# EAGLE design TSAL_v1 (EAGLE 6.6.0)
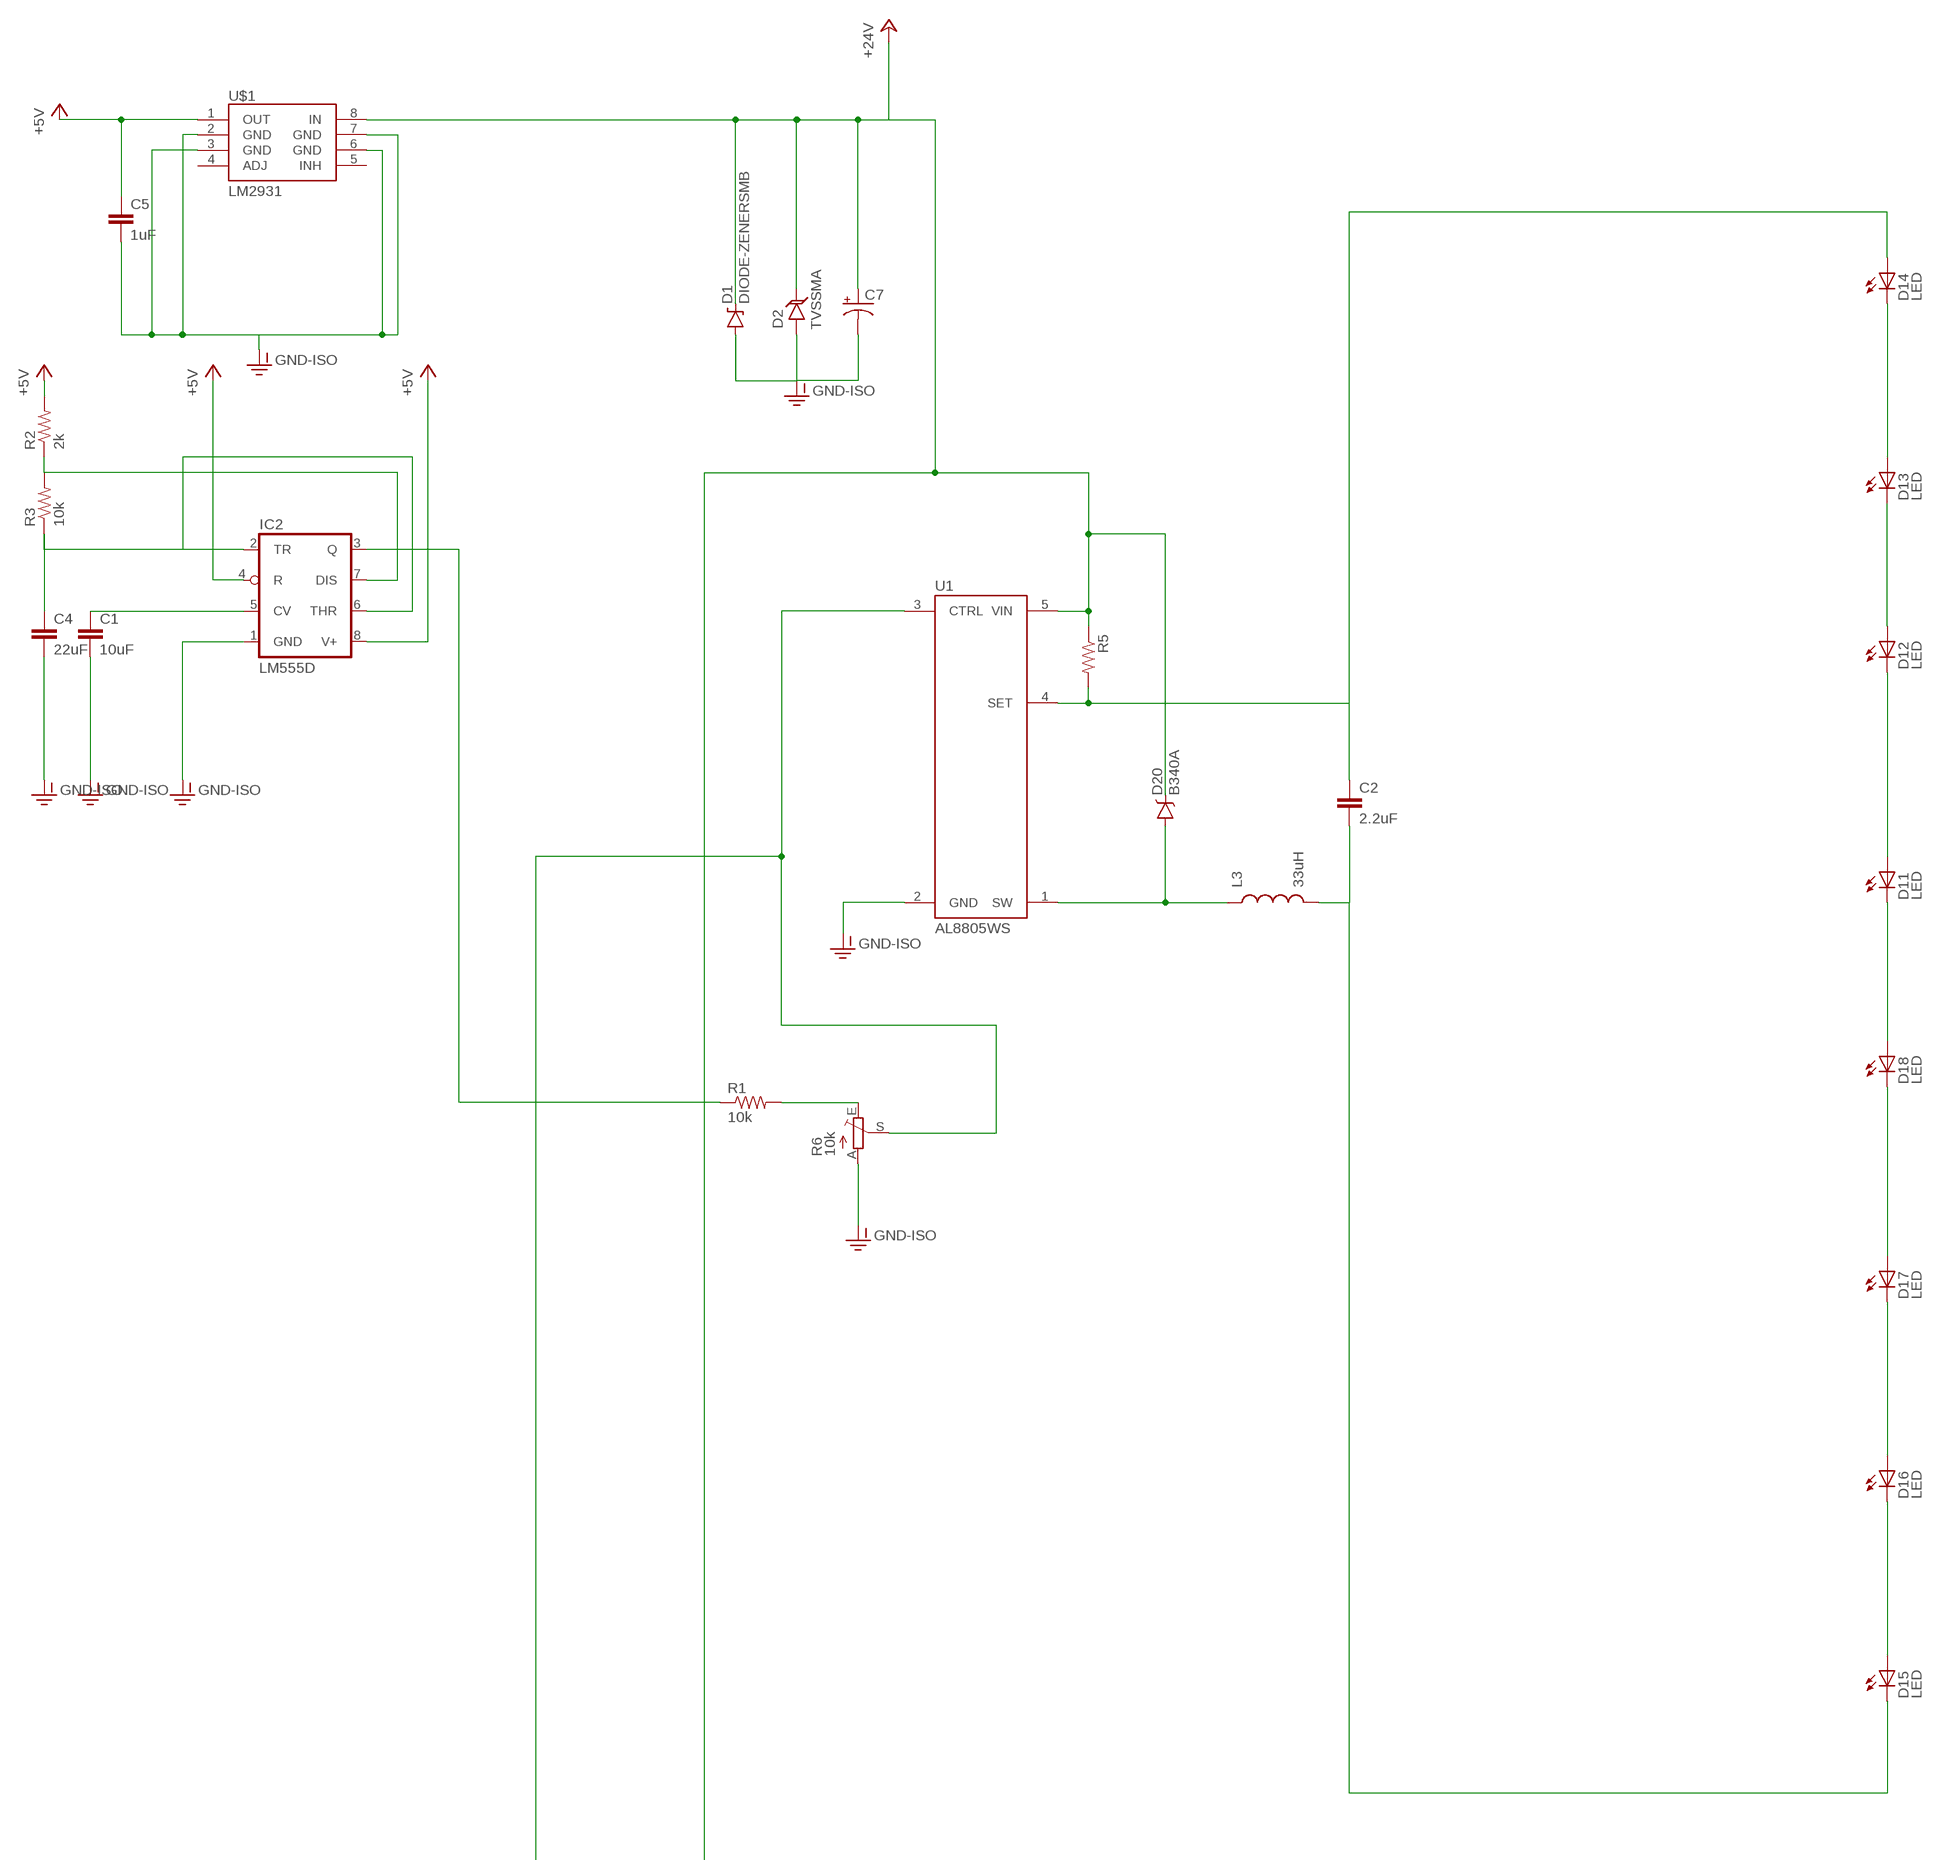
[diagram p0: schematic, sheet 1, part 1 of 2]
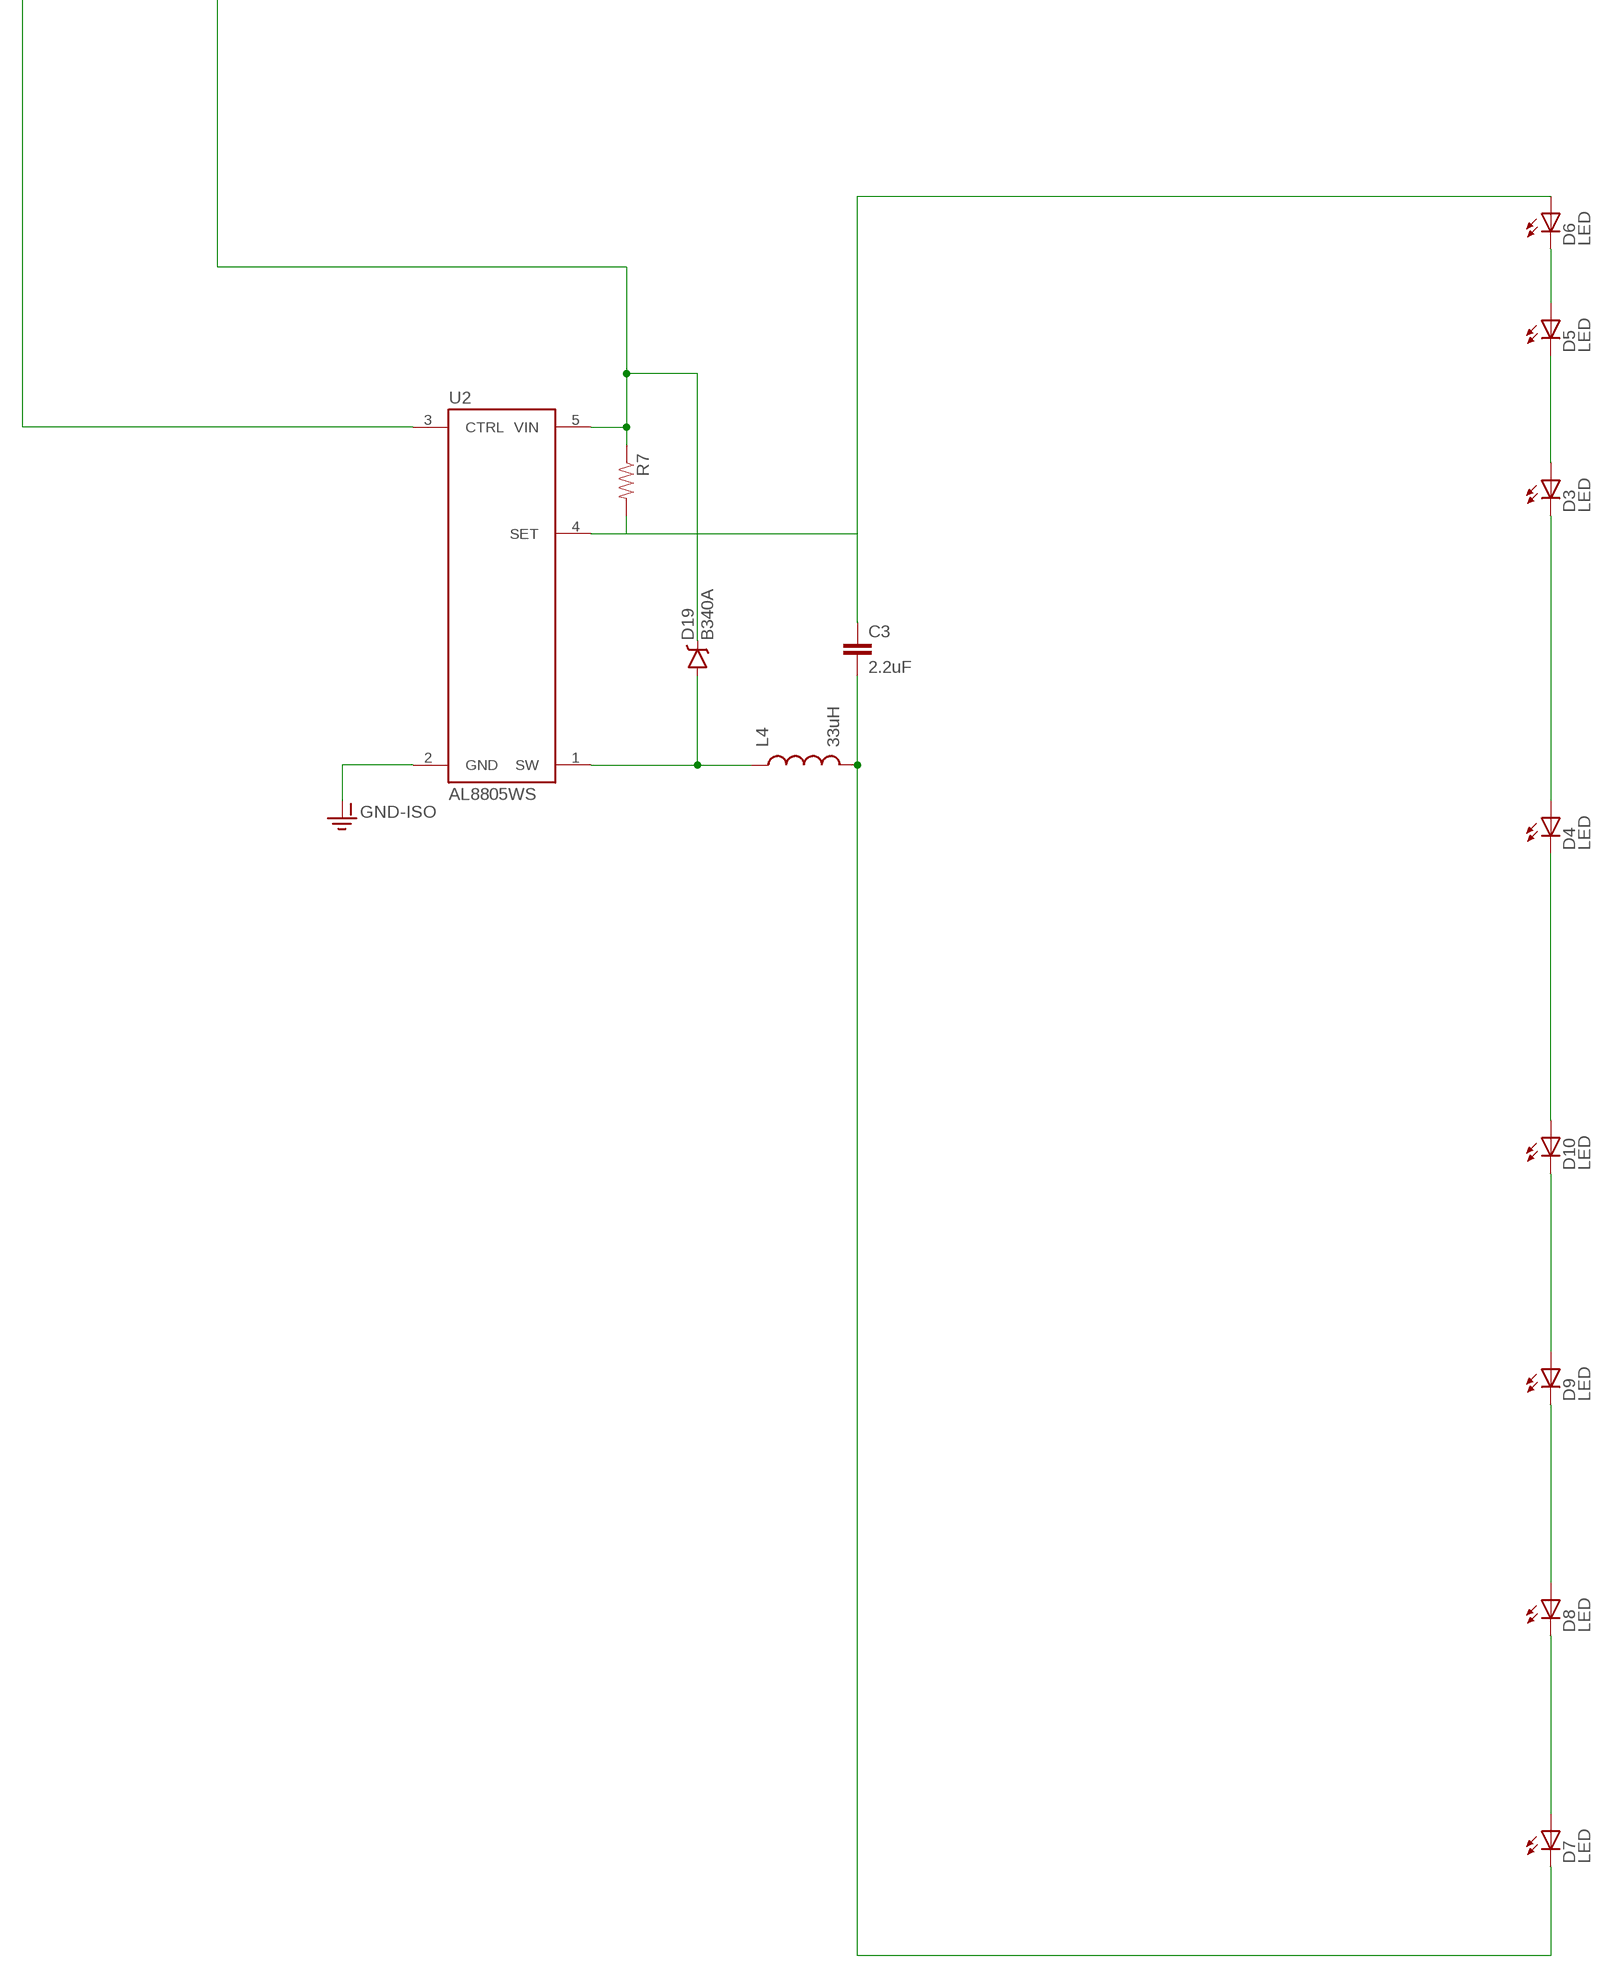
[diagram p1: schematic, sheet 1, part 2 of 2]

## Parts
C1  10uF  CAP0805  [0805]
C2  2.2uF  CAP0805  [0805]
C3  2.2uF  CAP0805  [0805]
C4  22uF  CAP0805  [0805]
C5  1uF  CAP0805  [0805]
C7  CAP_POL6032  [EIA6032]
D1  DIODE-ZENERSMB  [SMB-DIODE]
D2  TVSSMA  [SMA-DIODE]
D3  LED  [LED-SM]
D4  LED  [LED-SM]
D5  LED  [LED-SM]
D6  LED  [LED-SM]
D7  LED  [LED-SM]
D8  LED  [LED-SM]
D9  LED  [LED-SM]
D10  LED  [LED-SM]
D11  LED  [LED-SM]
D12  LED  [LED-SM]
D13  LED  [LED-SM]
D14  LED  [LED-SM]
D15  LED  [LED-SM]
D16  LED  [LED-SM]
D17  LED  [LED-SM]
D18  LED  [LED-SM]
D19  B340A  DIODE-SCHOTTKY-B340A  [SMA-DIODE]
D20  B340A  DIODE-SCHOTTKY-B340A  [SMA-DIODE]
IC2  LM555D  [SO08]
L3  33uH  INDUCTORBOURNS_SRN6045  [SRN6045]
L4  33uH  INDUCTORBOURNS_SRN6045  [SRN6045]
R1  10k  RESISTOR0805-RES  [0805]
R2  2k  RESISTOR0805-RES  [0805]
R3  10k  RESISTOR0805-RES  [0805]
R5  RESISTOR0805-RES  [0805]
R6  10k  TRIM_EU-B25P  [B25P]
R7  RESISTOR0805-RES  [0805]
U1  AL8805WS  AL8805  [SOT23-5]
U2  AL8805WS  AL8805  [SOT23-5]
U$1  LM2931  [SO08]

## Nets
+5V: C5.1 IC2.4(R) IC2.8(V+) R2.2 U$1.1(OUT)
+24V: C7.P$1(+) D1.C D2.C D19.C D20.C R5.1 R7.1 U1.5(VIN) U2.5(VIN) U$1.8(IN)
GND-ISO: C1.2 C4.2 C5.2 C7.P$2(-) D1.A D2.A IC2.1(GND) R6.A U1.2(GND) U2.2(GND) U$1.2(GND) U$1.3(GND) U$1.6(GND) U$1.7(GND)
N$1: C3.1 D6.A R7.2 U2.4(SET)
N$2: R6.S U1.3(CTRL) U2.3(CTRL)
N$3: D3.C D4.A
N$4: C1.1 IC2.5(CV)
N$5: IC2.7(DIS) R2.1 R3.2
N$6: IC2.3(Q) R1.1
N$7: D19.A L4.1 U2.1(SW)
N$8: C2.1 D14.A R5.2 U1.4(SET)
N$9: D13.A D14.C
N$10: C4.1 IC2.2(TR) IC2.6(THR) R3.1
N$11: D3.A D5.C
N$12: D12.A D13.C
N$13: D11.A D12.C
N$14: C3.2 D7.C L4.2
N$15: D11.C D18.A
N$16: D17.A D18.C
N$17: D5.A D6.C
N$18: D7.A D8.C
N$19: C2.2 D15.C L3.2
N$20: D8.A D9.C
N$21: D4.C D10.A
N$22: D9.A D10.C
N$23: D16.A D17.C
N$24: D15.A D16.C
N$26: D20.A L3.1 U1.1(SW)
N$27: R1.2 R6.E
Unconnected: U$1.4(ADJ) U$1.5(INH)

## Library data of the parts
C1-C5 = SparkFun-Capacitors:CAP: Capacitor
C7 = SparkFun-Capacitors:CAP_POL: Capacitor Polarized
D1 = SparkFun-DiscreteSemi:DIODE-ZENER: Zener Diode
D2 = SparkFun-DiscreteSemi:TVS: Transient voltage suppressor- prevents ESD on inputs.
D3-D18 = FSAE Eletric:LED
D19 D20 = SparkFun-DiscreteSemi:DIODE-SCHOTTKY: Schottky diodes in SFE's production catalog; PROD_ID: DIO-09886
IC2 = adafruit:*555: TIMER Changed DIP package to have round (not oval) pin pads http://www.ladyada.net/library/pcb/eaglelibrary.html
L3 L4 = SparkFun-Passives:INDUCTOR: Inductors; PROD_ID: NDUC-11627
R1-R3 R5 R7 = SparkFun-Passives:RESISTOR: Resistor
R6 = pot:TRIM_EU-: POTENTIOMETER
U1 U2 = SparkFun-PowerIC:AL8805: Constant current LED driver PWM-able 1MHz switch freq 6V-36V Up to 1A LED current; PROD_ID: IC-11626
U$1 = SparkFun-PowerIC:LM2931: LDO regulator with reverse battery protection- very durable!

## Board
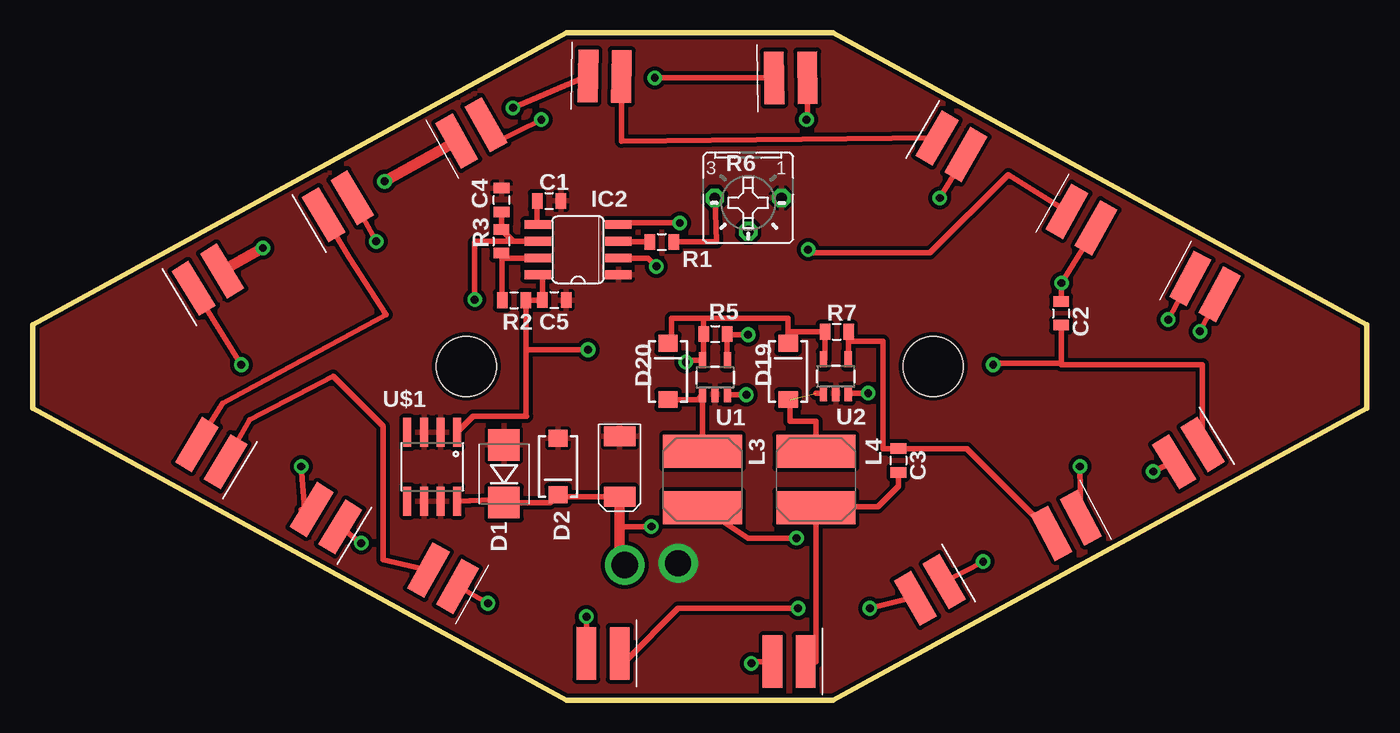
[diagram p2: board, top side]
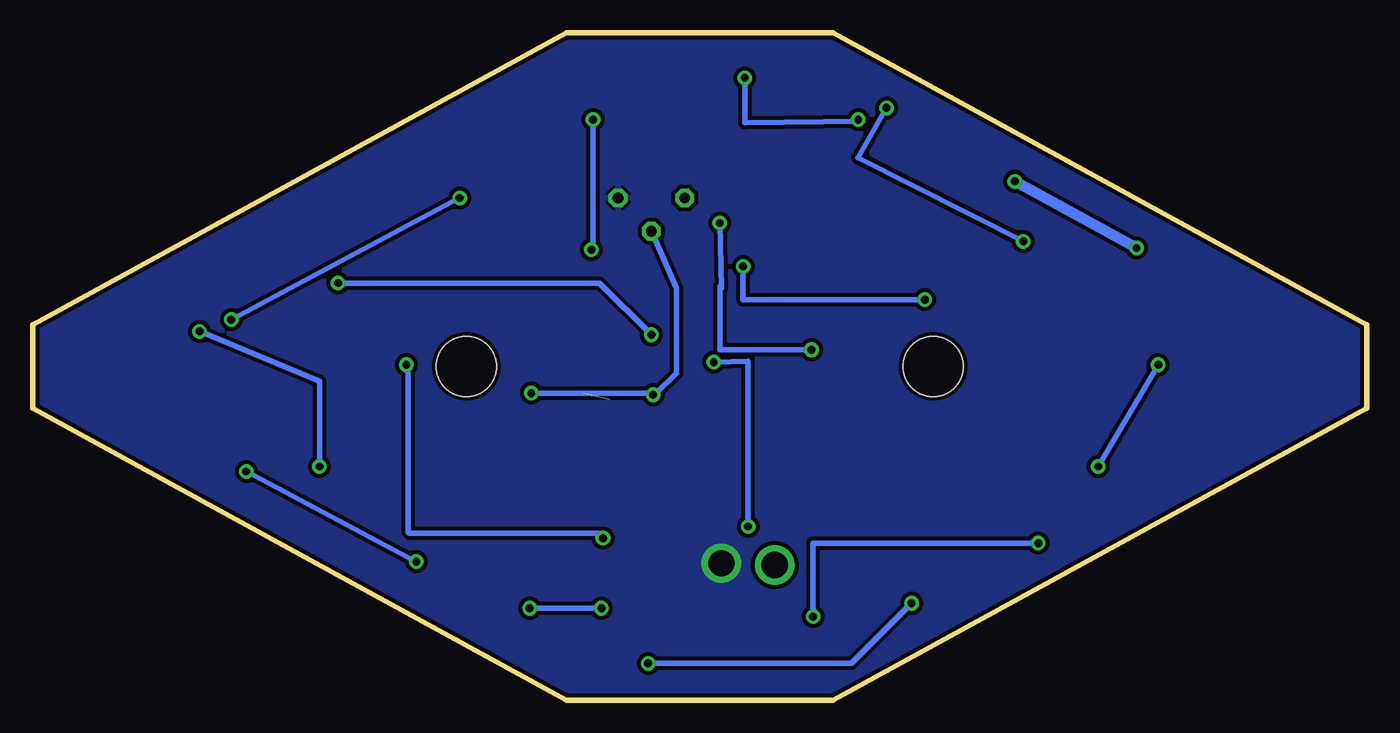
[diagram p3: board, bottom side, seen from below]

Size 101.6 x 50.8 mm. Coordinates in mm from the lower left corner, seen from the top.
Outline: 0,22.22 0,28.57 40.64,50.8 60.96,50.8 101.6,28.57 101.6,22.22 60.96,0 40.64,0 0,22.22
Copper layers (1*16): Top 0.035mm / dielectric 1.5mm / Bottom 0.035mm
Design rules "SparkFun": minimum track width 8mil, minimum drill 20mil, track to track 8mil, track to pad 8mil, pad to pad 8mil, via to via 8mil, smd to smd 8mil, copper to edge 10mil, drill to drill 8mil, minimum pad ring 12mil, minimum via ring 10mil, stop-mask expansion 4mil, vias tented up to drill 25mil, thermal gap 10mil
Holes 4.57 mm at 33.02,25.4 68.58,25.4

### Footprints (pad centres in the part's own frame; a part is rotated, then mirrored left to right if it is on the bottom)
0805 = smd 0.8 x 1.2: 1 -0.9,0; 2 0.9,0
EIA6032 = smd 1.5 x 2.4: P$1 -2.3,0; P$2 2.3,0
SMB-DIODE = smd 2.4 x 2.4: A 2.2,0; C -2.2,0
SMA-DIODE = smd 1.27 x 1.47: A -2.15,0; C 2.15,0
LED-SM = smd 1.5 x 4: A 1.27,0; C -1.27,0
SO08 = smd 0.66 x 2.032: 1 -1.905,-3.073; 2 -0.635,-3.073; 3 0.635,-3.073; 4 1.905,-3.073; 5 1.905,3.073; 6 0.635,3.073; 7 -0.635,3.073; 8 -1.905,3.073
SRN6045 = smd 2.5 x 6: 1 -2.175,-0.175; 2 2.125,-0.175
B25P = drill 0.813 octagon: A -2.54,0; E 2.54,0; S 0,2.54
SOT23-5 = smd 0.55 x 1.2: 1 -0.95,-1.3; 2 0,-1.3; 3 0.95,-1.3; 4 0.95,1.3; 5 -0.95,1.3
SO08' = smd 0.61 x 2.21: 1 -1.905,-2.616; 2 -0.635,-2.616; 3 0.635,-2.616; 4 1.905,-2.616; 5 1.905,2.616; 6 0.635,2.616; 7 -0.635,2.616; 8 -1.905,2.616

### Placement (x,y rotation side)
C1  39.32,38 0 top
C2  78.33,29.44 270 top
C3  65.94,18.24 270 top
C4  35.71,38.07 90 top
C5  39.73,30.45 0 top
C7  44.7,17.78 90 top
D1  35.89,17.22 90 top
D2  40.01,17.78 270 top
D3  69.98,42.16 330 top
D4  43.56,47.5 359.1 top
D5  89.28,31.5 331.7 top
D6  78.71,13.28 207.9 top
D7  57.61,2.92 180.1 top
D8  31.24,9.27 150.7 top
D9  13.59,18.8 149.1 top
D10  23.24,37.59 30.7 top
D11  13.34,32 31.4 top
D12  33.4,43.18 29.4 top
D13  57.73,47.37 0.7 top
D14  79.88,36.58 330.5 top
D15  88.01,18.8 211.4 top
D16  68.33,8.38 210.2 top
D17  43.43,3.56 179.9 top
D18  22.33,13.84 148.7 top
D19  57.53,25.02 90 top
D20  48.39,25.02 90 top
IC2  41.53,34.29 90 top
L3  51.18,16.76 270 top
L4  59.82,16.76 270 top
R1  47.9,34.87 0 top
R2  36.65,30.43 0 top
R3  35.69,34.92 270 top
R5  51.99,27.86 0 top
R6  54.48,38.23 180 top
R7  61.24,28.04 0 top
U1  51.97,24.56 0 top
U2  61.16,24.64 0 top
U$1  LM2931  [SO08']  30.43,17.75 180 top

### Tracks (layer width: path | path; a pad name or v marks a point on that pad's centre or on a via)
+5V  (via drill 0.6)
  Top 0.406: U$1.1 33.55,21.59 37.59,21.59 37.55,21.63 37.55,26.92 | 37.55,26.92 R2.2 37.58,30.45 C5.1 38.83,32.38 IC2.8 | IC2.4 44.73,36.32 v49.28,36.32 | v42.29,26.67 37.81,26.67 arc-90 37.55,26.92
  Bottom 0.406: v49.28,36.32 49.15,31.37 49.28,31.37 | 49.28,31.37 49.28,31.5 | 49.28,31.37 49.28,26.67 v42.29,26.67
+24V  (via drill 0.6 pad 0.25, 2)
  Top 0.406: 51.09,29.08 48.64,29.08 48.64,27.17 D20.C | 51.09,29.08 R5.1 51.09,25.86 U1.5 50.25,25.86 v49.73,25.73 | 51.09,29.08 57.53,29.08 57.53,28.04 | D19.C 57.53,28.04 | 57.53,28.04 R7.1 60.34,25.94 U2.5 | U$1.8 33.25,15.17 36.74,15.3 36.74,15.02 | v47.12,13.21 44.7,13.21 C7.P$1 40.16,15.48 D2.C 39.4,15.02 36.74,15.02 | D1.C 36.74,15.02
  Top 0.813: v45.09,10.29 44.7,10.67 C7.P$1
  Bottom 0.406: v49.73,25.73 47.12,25.78 v47.12,13.21
GND-ISO  (via drill 2)
  other vias: 49.15,10.41
  pour Top (isolate 0.305): 40.51,50.55 60.83,50.55 101.47,28.7 101.47,22.1 60.83,0.25 41.02,0.25 0.38,22.61 0.38,28.7
  pour Bottom (isolate 0.305): 40.51,51.05 60.83,51.05 101.47,28.7 101.47,22.1 60.83,-0.25 40.51,-0.25 -0.13,22.1 -0.13,28.7
N$1
  Top 0.406: U2.4 62.13,27.06 | 62.13,27.06 R7.2 | 62.13,27.06 62.13,27.3 64.77,27.3 64.77,19.14 C3.1 71.14,19.14 D6.A
N$2  (via drill 0.6)
  Top 0.406: U2.3 63.63,23.34 v63.63,23.37 | v54.36,23.24 53.09,23.24 | 53.09,23.24 52.92,23.24 U1.3 52.92,23.34 52.99,23.34 53.09,23.24
  Bottom 0.406: v63.63,23.37 54.36,23.37 v54.36,23.24 54.23,23.24 52.58,24.89 52.58,31.37 R6.S
N$3
  Top 0.406: D3.C 44.83,42.55 D4.A
N$4
  Top 0.406: IC2.5 38.42,36.23 C1.1
N$5
  Top 0.406: 35.69,30.49 R2.1 35.75,33.27 35.75,33.66 | 35.75,33.66 IC2.7 | R3.2 35.75,34.02 35.75,33.66
N$6
  Top 0.406: IC2.3 44.65,34.87 R1.1
N$7  (1 unrouted)
  Top 0.406: U2.1 59.64,23.34 | L4.1 59.64,21.21 57.66,21.21 57.66,22.87 D19.A
N$8  (via drill 0.6 pad 0.25)
  Top 0.406: U1.4 52.89,25.89 R5.2 52.95,27.81 v54.48,27.81 | C2.1 v78.36,31.75 D14.A
  Bottom 0.406: v54.48,27.81 58.42,31.75 v78.36,31.75
N$9  (via drill 0.6 pad 0.25)
  Top 0.406: D14.C 74.3,40 68.33,34.04 58.8,34.04 v59.05,34.29 | v58.93,44.2 59,44.27 D13.A
  Bottom 0.406: v59.05,34.29 58.93,34.42 v58.93,44.2
N$10  (via drill 0.6)
  Top 0.406: C4.1 35.71,35.82 R3.1 36.59,34.92 IC2.6 33.78,34.92 33.78,34.8 33.66,34.8 v33.66,30.48 | v47.5,33.02 46.86,33.66 IC2.2
  Bottom 0.406: v47.5,33.02 47.5,30.48 v33.66,30.48
N$11  (via drill 0.6 pad 0.25)
  Top 0.406: D5.C v86.49,28.96 | v69.09,38.23 D3.A
  Bottom 0.406: v86.49,28.96 v69.09,38.23
N$12  (via drill 0.6 pad 0.25)
  Top 0.406: D13.C 56.45,47.37 v47.37,47.37 | v38.73,44.2 35.18,42.42 D12.A
  Bottom 0.406: v47.37,47.37 47.37,43.94 38.35,44.07 v38.73,44.2
N$13  (via drill 0.6)
  Top 0.813: D12.C v26.8,39.5 | v17.53,34.42 D11.A
  Bottom 0.813: v26.8,39.5 v17.53,34.42
N$14
  Top 0.406: D7.C 59.64,2.92 L4.2 60.69,14.73 64.39,14.73 65.94,16.28 C3.2
N$15  (via drill 0.6)
  Top 0.406: 20.45,14.5 20.7,14.5 | 20.7,14.5 D18.A | D11.C v15.88,25.53 | v20.45,17.78 20.7,14.5
  Bottom 0.406: v15.88,25.53 v20.45,17.78
N$16  (via drill 0.6)
  Top 0.406: D18.C v25.02,11.94 | v42.16,6.35 D17.A
  Bottom 0.406: v25.02,11.94 42.16,11.94 v42.16,6.35
N$17  (via drill 0.6 pad 0.25)
  Top 0.406: D6.C v79.76,17.78 | v88.9,28.07 D5.A
  Bottom 0.406: v79.76,17.78 79.76,24.26 v88.9,28.07
N$18  (via drill 0.6)
  Top 0.406: D8.C v34.67,7.37 | v54.74,2.79 54.86,2.92 D7.A
  Bottom 0.406: v34.67,7.37 39.24,2.79 v54.74,2.79
N$19  (via drill 0.6)
  Top 0.406: D15.C 89.09,25.53 78.36,25.53 78.36,25.65 | 78.36,25.65 78.36,28.54 C2.2 | L3.2 54.47,12.32 v58.17,12.32 | v73.15,25.53 73.28,25.65 78.36,25.65
  Bottom 0.406: v58.17,12.32 58.55,12.7 72.9,12.7 73.02,12.83 73.02,25.65 v73.15,25.53
N$20
  Top 0.406: D9.C 16.51,21.34 22.86,24.64 26.67,20.83 26.67,10.67 D8.A
N$21  (via drill 0.6 pad 0.25)
  Top 0.406: D4.C v36.58,45.09 | v26.16,34.92 D10.A
  Bottom 0.406: v36.58,45.09 38.73,41.27 v26.16,34.92
N$22
  Top 0.406: D10.C 24.13,33.66 26.92,29.34 14.48,22.61 D9.A
N$23  (via drill 0.6)
  Top 0.406: D17.C 45.22,3.04 49.16,6.98 v58.29,6.98 | v63.75,6.98 66.8,7.74 D16.A
  Bottom 0.406: v58.29,6.98 v63.75,6.98
N$24  (via drill 0.6)
  Top 0.406: D16.C v72.39,10.54 | v85.34,17.4 D15.A
  Bottom 0.406: v72.39,10.54 v85.34,17.4
N$26
  Top 0.406: D20.A 50.63,22.87 U1.1 51.02,20.47 L3.1
N$27
  Top 0.406: R1.2 52.07,34.87 R6.E

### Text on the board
_tsilk: R6 | 3 | 1 | C1 | IC2 | C4 | R3 | R1 | C2 | R5 | R7 | R2 | C5 | U$1 | D20 | D19 | U1 | U2 | L3 | L4 | C3 | D2 | D1

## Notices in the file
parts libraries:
SparkFun-PowerIC: Licensing: Creative Commons ShareAlike 4.0 International - https://creativecommons.org/licenses/by-sa/4.0
